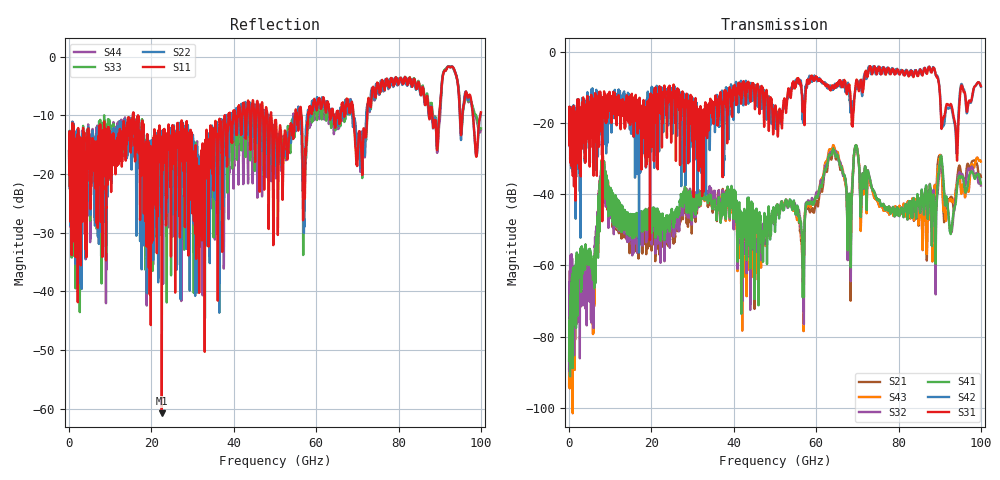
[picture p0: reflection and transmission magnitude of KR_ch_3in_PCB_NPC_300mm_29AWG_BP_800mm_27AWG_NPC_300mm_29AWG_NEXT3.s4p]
# GHz S RI R 45
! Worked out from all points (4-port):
!   4000 points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, 25 MHz to 100 GHz, reference 45 ohm
!   strongest paths, dB at 25 MHz, 25.02 GHz, 50.02 GHz, 75.03 GHz, 100 GHz:
!     S31: -20.7, -14.9, -15.8, -5.1, -9.6
!     S42: -20.6, -18.0, -18.0, -4.3, -9.8
!     S41: -86.8, -45.6, -50.6, -41.7, -37.0
!     S32: -88.7, -46.4, -47.4, -41.7, -37.5
!     S43: -89.3, -46.9, -46.1, -42.2, -30.8
!     S21: -93.8, -49.8, -47.2, -42.1, -35.1
!   lowest |S11| = -60.8 dB at 22.52 GHz (marker M1), VSWR 1.00, Z = 44.9 - j0.00886 ohm
!   |S11| at or under -10 dB: start of sweep to 15.52 GHz; 15.63 GHz to 38.73 GHz (23.1 GHz wide, 85 % of centre); 49.11 GHz to 54.96 GHz (5.845 GHz wide, 11.2 % of centre)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
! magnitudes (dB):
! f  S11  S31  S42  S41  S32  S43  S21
! 25 MHz  -16.1  -20.7  -20.6  -86.8  -88.7  -89.3  -93.8
! 5.9 GHz  -14.2  -20.4  -19.1  -64.0  -72.5  -78.9  -74.7
! 8.025 GHz  -19.6  -25.9  -26.6  -31.6  -31.9  -31.0  -32.4
! 22.52 GHz  -60.8  -23.3  -11.1  -48.4  -52.8  -48.9  -52.5
! 56.67 GHz  -16.7  -14.8  -19.0  -59.0  -59.0  -60.0  -58.1
! 63.85 GHz  -9.2  -9.6  -10.1  -28.4  -28.4  -27.4  -29.3
! 100 GHz  -9.5  -9.6  -9.8  -37.0  -37.5  -30.8  -35.1
